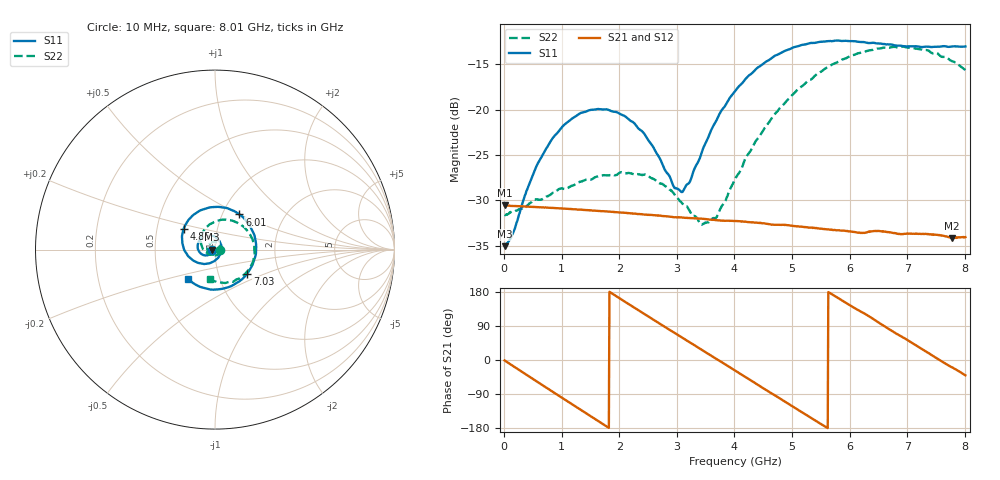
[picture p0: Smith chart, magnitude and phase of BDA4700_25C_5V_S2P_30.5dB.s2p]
!Agilent Technologies,E5071B,MY42404982,A.09.10
!Date: Mon Oct 20 13:41:58 2025
!Data & Calibration Information:
!Freq	S11:SOLT2(ON)	S21:SOLT2(ON)	S12:SOLT2(ON)	S22:SOLT2(ON)
# Hz S RI R 50
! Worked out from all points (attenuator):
!   801 points, 10 MHz to 8.01 GHz, reference 50 ohm
!   highest |S21| = -30.56 dB at 20 MHz (marker M1); lowest = -34.2 dB at 7.78 GHz (marker M2)
!   lowest |S11| = -35.1 dB at 10 MHz (marker M3), VSWR 1.04, Z = 48.3 - j0.0942 ohm
!   |S11| at or under -10 dB: start of sweep to end of sweep
!   |S22| runs from -32.7 to -13.0 dB; largest |S21 - S12| = 0.00026
!   S11 on the Smith chart (normalised r, x): 10 MHz: 0.97, -0.00; 4.85 GHz: 0.69, +0.16; 6.01 GHz: 1.20, +0.50; 7.03 GHz: 1.37, -0.39; 8.01 GHz: 0.70, -0.25
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1e7  -0.0176 -0.000976  0.0296 -0.000606  0.0297 -0.000665  0.0263 -0.000841
2e7  -0.0179 -0.00169  0.0296 -0.00109  0.0296 -0.0012  0.0262 -0.00111
1.6e8  -0.0185 -0.00987  0.0283 -0.00824  0.0283 -0.00823  0.0264 -0.00758
4.3e8  -0.0287 -0.0253  0.0213 -0.0199  0.0213 -0.0199  0.0196 -0.0227
7e8  -0.0487 -0.0324  0.01 -0.027  0.01 -0.027  0.00598 -0.0321
1.35e9  -0.0961 0.00641  -0.0193 -0.0204  -0.0193 -0.0204  -0.036 -0.0179
2.08e9  -0.0512 0.0774  -0.0246 0.0111  -0.0246 0.0112  -0.0298 0.0334
2.68e9  0.023 0.0504  -0.0037 0.0258  -0.00368 0.0258  0.0126 0.0375
2.95e9  0.0354 0.012  0.0077 0.0243  0.00769 0.0243  0.0251 0.0235
3.1e9  0.0333 -0.0117  0.0133 0.0216  0.0133 0.0216  0.028 0.0116
3.41e9  0.00609 -0.0549  0.0219 0.0122  0.022 0.0122  0.0205 -0.0114
3.54e9  -0.0128 -0.0684  0.0238 0.00713  0.0238 0.00703  0.013 -0.02
3.7e9  -0.0427 -0.0779  0.0245 0.000686  0.0246 0.000593  -0.000523 -0.0259
4.01e9  -0.1056 -0.0688  0.0216 -0.0113  0.0216 -0.0113  -0.0321 -0.0258
4.85e9  -0.1749 0.1144  -0.00687 -0.0221  -0.00679 -0.0222  -0.0757 0.0751
5.35e9  -0.0743 0.2212  -0.0202 -0.00959  -0.0201 -0.00963  -0.0155 0.1477
6.01e9  0.1361 0.196  -0.0173 0.0125  -0.0173 0.0125  0.1331 0.1464
6.68e9  0.2284 -0.0146  0.003 0.0209  0.00305 0.0209  0.2198 0.000351
7.03e9  0.1795 -0.1333  0.0132 0.016  0.0133 0.0158  0.1991 -0.0931
7.42e9  0.0595 -0.2136  0.02 0.00476  0.0199 0.00469  0.1228 -0.1655
7.78e9  -0.0768 -0.2095  0.0184 -0.00663  0.0185 -0.00669  0.026 -0.1831
8.01e9  -0.1495 -0.1657  0.0151 -0.0128  0.0151 -0.0128  -0.0299 -0.1623
